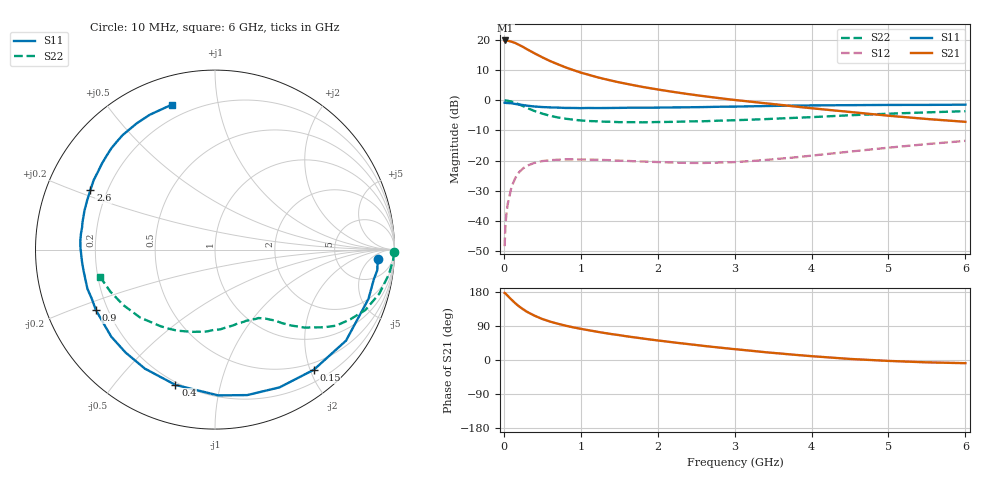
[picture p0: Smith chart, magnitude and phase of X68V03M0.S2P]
! SIEMENS Small Signal Semiconductors
! BFP193W
! Si NPN RF Bipolar Junction Transistor in SOT343
! VCE = 8 V  IC = 3 mA
! Common Emitter S-Parameters:  April 1994
# GHz  S  MA  R  50
!  f  S11  S21  S12  S22
! GHz  MAG  ANG  MAG  ANG  MAG  ANG  MAG  ANG
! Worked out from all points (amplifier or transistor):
!   40 points, 10 MHz to 6 GHz, reference 50 ohm
!   highest |S21| = 19.8 dB at 20 MHz (marker M1)
!   |S21| within 3 dB of that: start of sweep to 308 MHz
!   unconditionally stable (mu >= 1): 1.982 GHz to 4.711 GHz
!   at 200 MHz: K = 0.11, MSG = 21.1 dB, |S12| = -23.8 dB
!   at 1.5 GHz: K = 0.76, MSG = 13.0 dB, |S12| = -20.0 dB
!   at 6 GHz: K = 0.93, MSG = 3.2 dB, |S12| = -13.5 dB
!   S11 on the Smith chart (normalised r, x): 10 MHz: 15, -9; 150 MHz: 0.38, -2.06; 400 MHz: 0.19, -0.73; 900 MHz: 0.15, -0.23; 2.6 GHz: 0.14, +0.22; 6 GHz: 0.13, +0.74
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0.01  0.9077 -3.4  9.725 177.0  0.0038 87.3  0.9983 -0.8
0.02  0.9114 -7.2  9.786 175.7  0.0079 85.0  0.9943 -3.3
0.05  0.898 -17.8  9.698 169.4  0.0189 80.5  0.9797 -7.9
0.1  0.8889 -34.8  9.335 159.2  0.0366 70.9  0.9478 -15.0
0.15  0.8668 -50.6  8.865 149.6  0.0516 62.7  0.9028 -21.9
0.2  0.8477 -64.9  8.24 141.1  0.0643 55.5  0.8486 -27.2
0.25  0.8302 -77.5  7.642 134.0  0.0741 49.4  0.7973 -32.1
0.3  0.8125 -88.7  7.017 127.3  0.0818 44.1  0.7453 -35.5
0.4  0.7855 -106.3  5.98 116.8  0.0916 35.6  0.6608 -41.1
0.5  0.7697 -120.5  5.139 108.2  0.0979 29.7  0.5991 -44.9
0.6  0.7597 -131.0  4.466 101.4  0.101 25.2  0.5517 -47.8
0.7  0.7546 -140.0  3.954 95.8  0.1031 21.9  0.5183 -49.7
0.9  0.7441 -153.1  3.169 86.3  0.1045 17.1  0.4753 -53.9
1.1  0.7436 -162.9  2.643 78.6  0.1036 14.2  0.4516 -57.6
1.3  0.7418 -171.1  2.259 71.6  0.102 12.5  0.441 -61.8
1.6  0.7497 179.2  1.865 62.4  0.0987 12.1  0.433 -67.9
2.2  0.759 163.4  1.374 46.6  0.0926 15.9  0.4375 -81.5
2.6  0.7694 154.5  1.166 37.2  0.0912 21.5  0.4478 -91.1
3.2  0.7918 142.6  0.948 24.7  0.0977 31.0  0.4751 -105.4
4.5  0.8278 121.7  0.638 2.8  0.1405 42.0  0.5631 -137.7
5.5  0.8358 111.3  0.488 -6.2  0.1871 40.5  0.6285 -158.2
6  0.843 106.5  0.438 -8.4  0.2119 38.5  0.6575 -166.5
